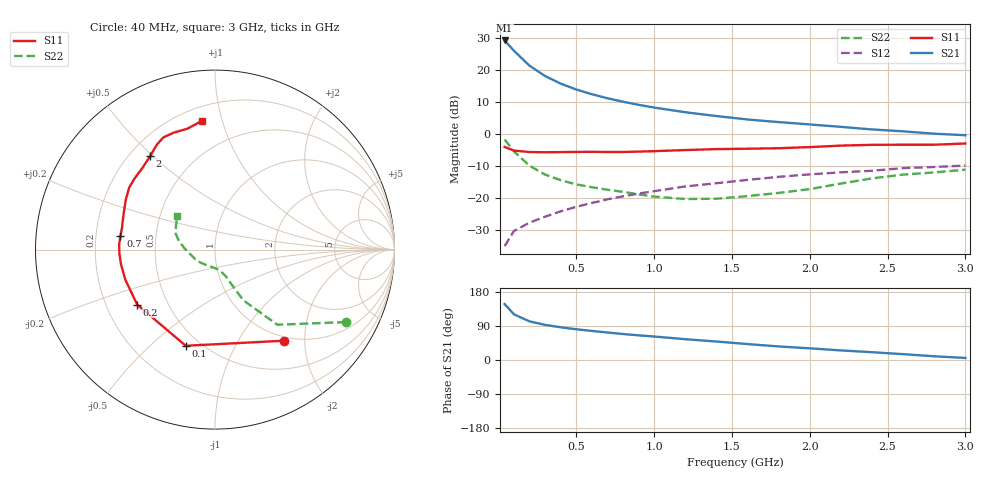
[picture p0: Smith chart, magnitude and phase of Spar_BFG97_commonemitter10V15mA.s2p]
! Filename:  BFG97E.S2P  Version:  2.0
! NXP part #: BFG97  Date: Jul 1990
! Bias condition: Vce=10V, Ic=15mA
#  MHz  S  MA  R  50
! Freq  S11  S21  S12  S22  !GUM [dB]
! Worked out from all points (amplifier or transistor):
!   21 points, 40 MHz to 3 GHz, reference 50 ohm
!   highest |S21| = 29.3 dB at 40 MHz (marker M1)
!   |S21| within 3 dB of that: start of sweep to 95.78 MHz
!   unconditionally stable (mu >= 1): 427.1 MHz to end of sweep
!   at 300 MHz: K = 0.89, MSG = 22.0 dB, |S12| = -25.7 dB
!   at 1 GHz: K = 1.15, MAG = 10.7 dB, |S12| = -17.7 dB
!   at 3 GHz: K = 1.05, MAG = 3.3 dB, |S12| = -9.7 dB
!   S11 on the Smith chart (normalised r, x): 40 MHz: 0.94, -1.60; 100 MHz: 0.42, -0.65; 200 MHz: 0.33, -0.29; 700 MHz: 0.31, +0.06; 2 GHz: 0.28, +0.49; 3 GHz: 0.29, +0.86
40  0.638 -52.7  29.33 147.6  0.018 68.5  0.833 -29.0
100  0.56 -106.9  20.23 120.6  0.031 53.4  0.544 -50.3
200  0.531 -144.7  11.84 101.9  0.042 52.1  0.324 -60.8
300  0.527 -161.3  8.17 92.7  0.052 54.8  0.236 -63.6
400  0.53 -170.8  6.218 86.3  0.063 57.9  0.193 -65.7
500  0.533 -177.5  5.026 81.1  0.074 59.5  0.166 -67.3
600  0.535 177.0  4.252 76.7  0.085 60.7  0.15 -69.4
700  0.532 171.9  3.674 72.6  0.097 62.1  0.137 -72.4
800  0.532 167.0  3.243 68.6  0.108 61.9  0.127 -75.5
900  0.539 162.4  2.901 65.1  0.119 62.0  0.116 -79.1
1000  0.548 158.1  2.629 62.0  0.13 61.8  0.107 -85.7
1200  0.57 150.6  2.222 54.9  0.154 60.8  0.098 -102.3
1400  0.59 144.1  1.937 48.8  0.173 58.7  0.099 -121.2
1600  0.598 138.7  1.712 42.0  0.195 58.1  0.109 -138.4
1800  0.609 131.5  1.559 35.8  0.218 54.4  0.122 -153.5
2000  0.634 124.7  1.432 30.8  0.238 53.5  0.14 -169.6
2200  0.669 118.9  1.313 25.3  0.256 50.8  0.171 177.2
2400  0.688 114.6  1.197 20.6  0.271 49.9  0.206 166.8
2600  0.691 109.5  1.118 15.4  0.298 46.6  0.236 158.0
2800  0.691 102.8  1.027 9.8  0.31 42.2  0.255 148.5
3000  0.722 95.6  0.972 5.4  0.327 40.6  0.282 137.9
